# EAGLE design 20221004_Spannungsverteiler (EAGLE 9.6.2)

## Sheet 1 of 3: Anschlussklemmen
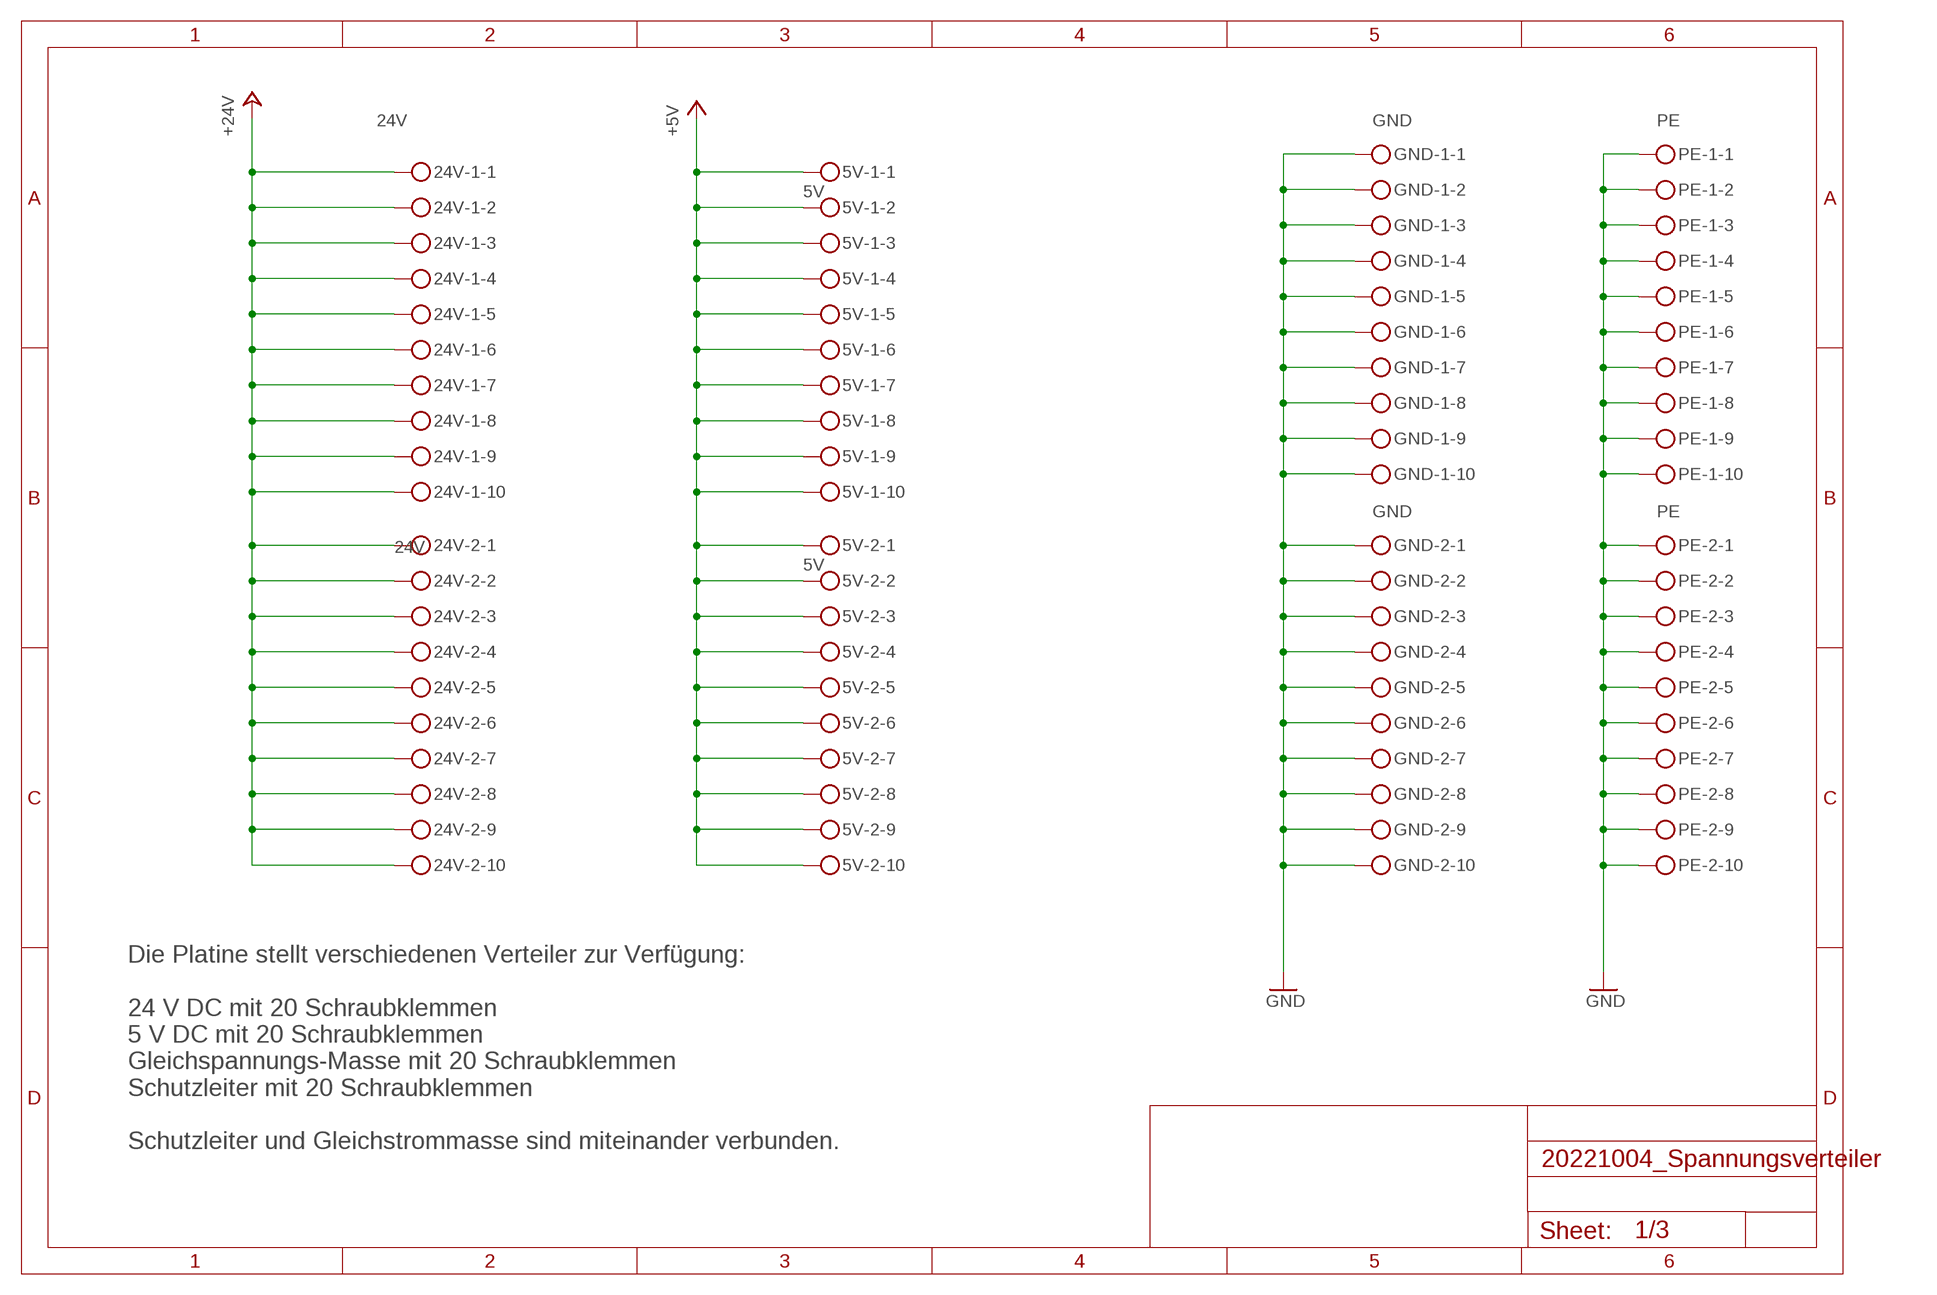
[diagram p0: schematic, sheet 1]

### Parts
5V-1  5V  MKDSN1,5/10-5,08  [MKDSN1,5/10-5,08]
5V-2  5V  MKDSN1,5/10-5,08  [MKDSN1,5/10-5,08]
24V-1  24V  MKDSN1,5/10-5,08  [MKDSN1,5/10-5,08]
24V-2  24V  MKDSN1,5/10-5,08  [MKDSN1,5/10-5,08]
GND-1  GND  MKDSN1,5/10-5,08  [MKDSN1,5/10-5,08]
GND-2  GND  MKDSN1,5/10-5,08  [MKDSN1,5/10-5,08]
PE-1  PE  MKDSN1,5/10-5,08  [MKDSN1,5/10-5,08]
PE-2  PE  MKDSN1,5/10-5,08  [MKDSN1,5/10-5,08]

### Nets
+5V: 5V-1.1 5V-1.2 5V-1.3 5V-1.4 5V-1.5 5V-1.6 5V-1.7 5V-1.8 5V-1.9 5V-1.10 5V-2.1 5V-2.2 5V-2.3 5V-2.4 5V-2.5 5V-2.6 5V-2.7 5V-2.8 5V-2.9 5V-2.10 ; also sheet 2,3
+24V: 24V-1.1 24V-1.2 24V-1.3 24V-1.4 24V-1.5 24V-1.6 24V-1.7 24V-1.8 24V-1.9 24V-1.10 24V-2.1 24V-2.2 24V-2.3 24V-2.4 24V-2.5 24V-2.6 24V-2.7 24V-2.8 24V-2.9 24V-2.10 ; also sheet 3
GND: GND-1.1 GND-1.2 GND-1.3 GND-1.4 GND-1.5 GND-1.6 GND-1.7 GND-1.8 GND-1.9 GND-1.10 GND-2.1 GND-2.2 GND-2.3 GND-2.4 GND-2.5 GND-2.6 GND-2.7 GND-2.8 GND-2.9 GND-2.10 PE-1.1 PE-1.2 PE-1.3 PE-1.4 PE-1.5 PE-1.6 PE-1.7 PE-1.8 PE-1.9 PE-1.10 PE-2.1 PE-2.2 PE-2.3 PE-2.4 PE-2.5 PE-2.6 PE-2.7 PE-2.8 PE-2.9 PE-2.10 ; also sheet 2,3

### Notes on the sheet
- Die Platine stellt verschiedenen Verteiler zur Verfügung:
  
  24 V DC mit 20 Schraubklemmen
  5 V DC mit 20 Schraubklemmen
  Gleichspannungs-Masse mit 20 Schraubklemmen
  Schutzleiter mit 20 Schraubklemmen
  
  Schutzleiter und Gleichstrommasse sind miteinander verbunden.

## Sheet 2 of 3: Schaltungen
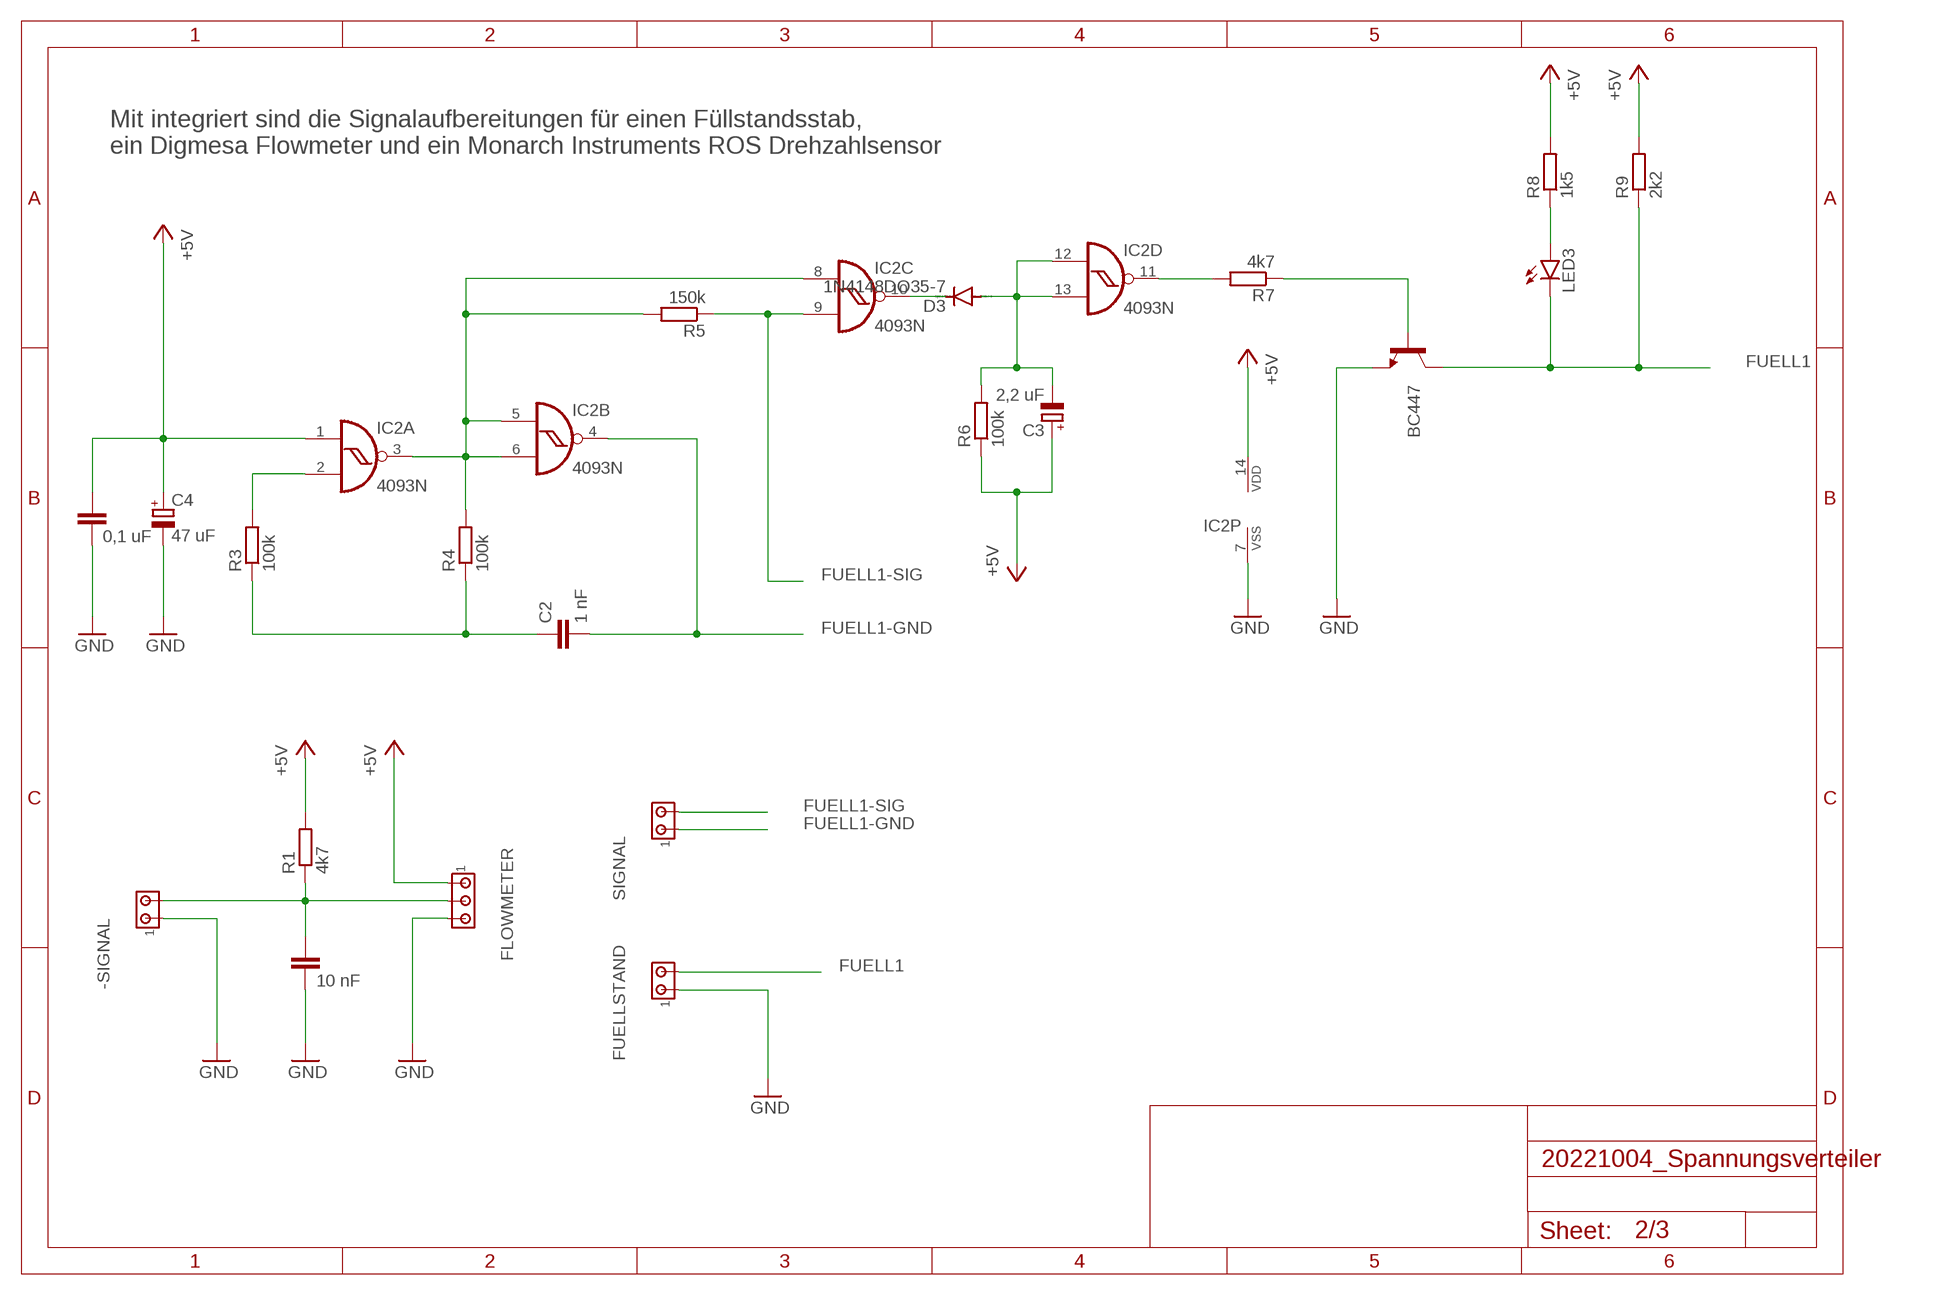
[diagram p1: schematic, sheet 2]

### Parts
-SIGNAL  MTA02-100  [10X02MTA]
C1  10 nF  C-EU050-024X044  [C050-024X044]
C2  1 nF  C-EU050-024X044  [C050-024X044]
C3  2,2 uF  CPOL-EUE2.5-7  [E2,5-7]
C4  47 uF  CPOL-EUE2.5-7  [E2,5-7]
C5  0,1 uF  C-EU050-024X044  [C050-024X044]
D3  1N4148DO35-7  [DO35-7]
FLOWMETER  MTA03-100  [10X03MTA]
FUELLSTAND  MTA02-100  [10X02MTA]
IC2  4093N  [DIL14]
LED3  LED3MM  [LED3MM]
Q1  BC447  [TO92-EBC]
R1  4k7  R-EU_0204/7  [0204/7]
R3  100k  R-EU_0204/7  [0204/7]
R4  100k  R-EU_0204/7  [0204/7]
R5  150k  R-EU_0204/7  [0204/7]
R6  100k  R-EU_0204/7  [0204/7]
R7  4k7  R-EU_0204/7  [0204/7]
R8  1k5  R-EU_0204/7  [0204/7]
R9  2k2  R-EU_0204/7  [0204/7]
SIGNAL  MTA02-100  [10X02MTA]

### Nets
+5V: C3.+ C4.+ C5.1 FLOWMETER.1 IC2.1(A:I0) IC2.14(P:VDD) R1.2 R6.1 R8.2 R9.2 ; also sheet 1,3
FUELL1: FUELLSTAND.2 LED3.K(C) Q1.C R9.1
FUELL1-GND: C2.2 IC2.4(B:O) SIGNAL.1
FUELL1-SIG: IC2.9(C:I1) R5.1 SIGNAL.2
GND: -SIGNAL.1 C1.2 C4.- C5.2 FLOWMETER.3 FUELLSTAND.1 IC2.7(P:VSS) Q1.E ; also sheet 1,3
N$2: -SIGNAL.2 C1.1 FLOWMETER.2 R1.1
N$3: IC2.2(A:I1) R3.2
N$4: IC2.3(A:O) IC2.5(B:I0) IC2.6(B:I1) IC2.8(C:I0) R4.2 R5.2
N$5: C2.1 R3.1 R4.1
N$6: D3.C IC2.10(C:O)
N$7: C3.- D3.A IC2.12(D:I0) IC2.13(D:I1) R6.2
N$8: IC2.11(D:O) R7.2
N$9: Q1.B R7.1
N$10: LED3.A R8.1

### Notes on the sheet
- Mit integriert sind die Signalaufbereitungen für einen Füllstandsstab, 
  ein Digmesa Flowmeter und ein Monarch Instruments ROS Drehzahlsensor

## Sheet 3 of 3: Spannungsregler
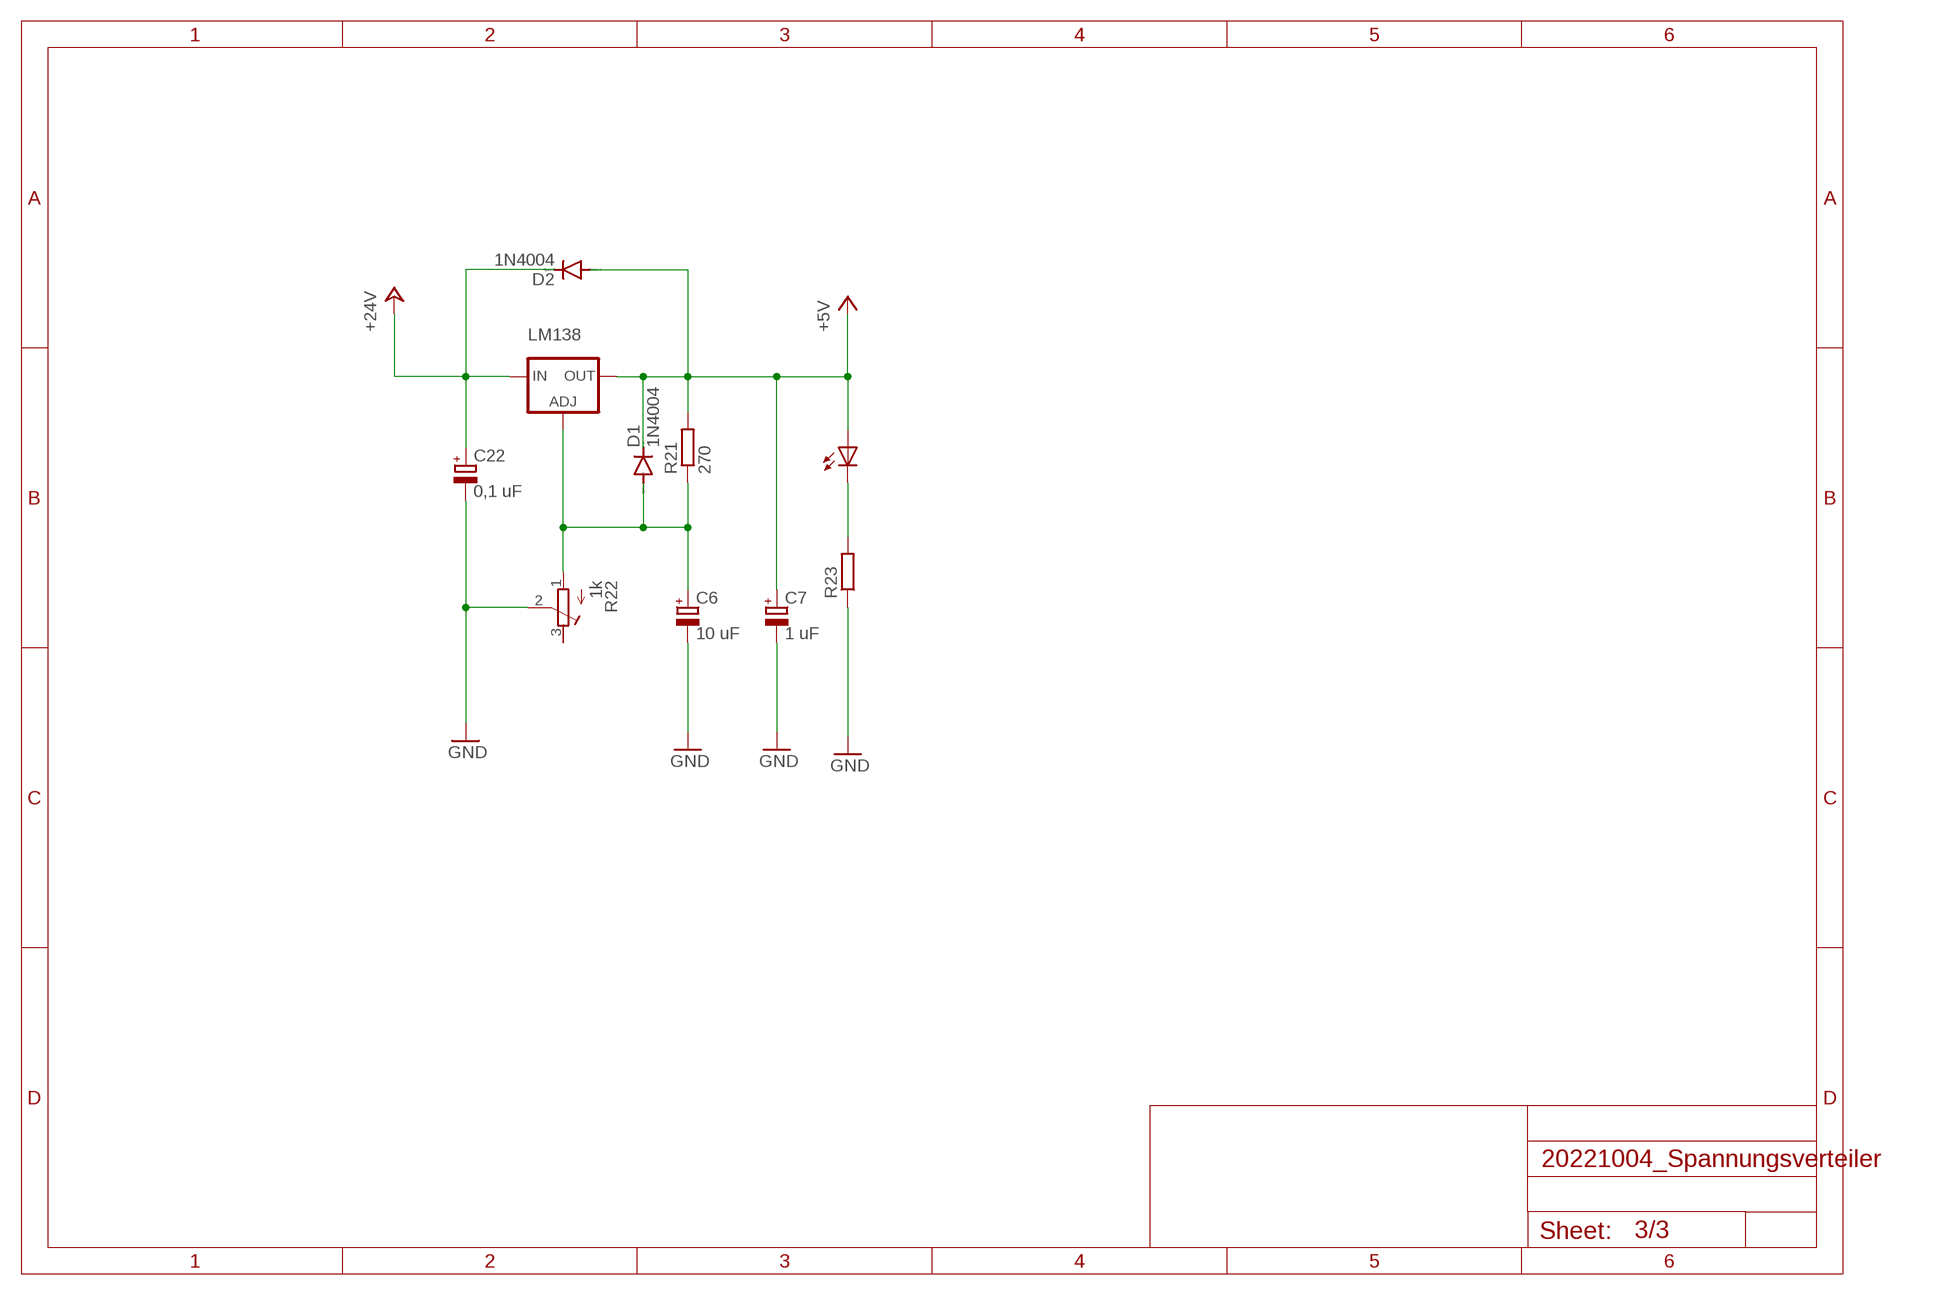
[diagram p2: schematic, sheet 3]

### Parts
C6  10 uF  CPOL-EUE2-5  [E2-5]
C7  1 uF  CPOL-EUE2-5  [E2-5]
C22  0,1 uF  CPOL-EUE2-5  [E2-5]
D1  1N4004  [DO41-10]
D2  1N4004  [DO41-10]
LED16  TLLG4400  [LED3MM]
LM138  LM138-TL  [TO220L1]
R21  270  R-EU_0204/7  [0204/7]
R22  1k  R-TRIMM64Y  [RTRIM64Y]
R23  R-EU_0204/7  [0204/7]

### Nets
+5V: C7.+ D1.C D2.A LED16.A LM138.2(OUT) R21.2 ; also sheet 1,2
+24V: C22.+ D2.C LM138.3(IN) ; also sheet 1
GND: C6.- C7.- C22.- R22.2(S) R23.1 ; also sheet 1,2
N$11: C6.+ D1.A LM138.1(ADJ) R21.1 R22.1(A)
N$14: LED16.K(C) R23.2
Unconnected: R22.3(E)

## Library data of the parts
5V-1 5V-2 24V-1 24V-2 GND-1 GND-2 PE-1 PE-2 = con-phoenix-508:MKDSN1,5/10-5,08: MKDSN 1,5/10-5,08 Printklemme Nennstrom: 13,5 A Nennspannung: 250 V Rastermaß: 5,08 mm Polzahl: 10 Anschlussart: Schraubanschluss Montage: Löten Anschlussrichtung Leiter/Platine: 0 ° Artikelnummer: 1729209 Source: http://eshop.phoenixcontact.com .. 1729209.pdf
-SIGNAL FUELLSTAND SIGNAL = con-amp:MTA02-100: AMP connector
C1 C2 C5 = resistor:C-EU: CAPACITOR, European symbol
C3 C4 C6 C7 C22 = resistor:CPOL-EU: POLARIZED CAPACITOR, European symbol
D1 D2 = diode:1N4004: DIODE
D3 = diode:1N4148: DIODE
FLOWMETER = con-amp:MTA03-100: AMP connector
IC2 = 40xx:4093: Quad 2-input NAND schmitt trigger
LED3 = led:LED: LED
LED16 = led:TLLG4400: Low Current (2mA) LED 3 mm Tinted Diffused Package color GREEN; MF: VISHAY SEMICONDUCTOR; OC_FARNELL: 1612435
LM138 = v-reg:LM138-TL: VOLTAGE REGULATOR
Q1 = transistor-npn:BC447*: NPN Transistor
R1 R3-R9 R21 R23 = resistor:R-EU_: RESISTOR, European symbol
R22 = resistor:R-TRIMM: Trimm resistor

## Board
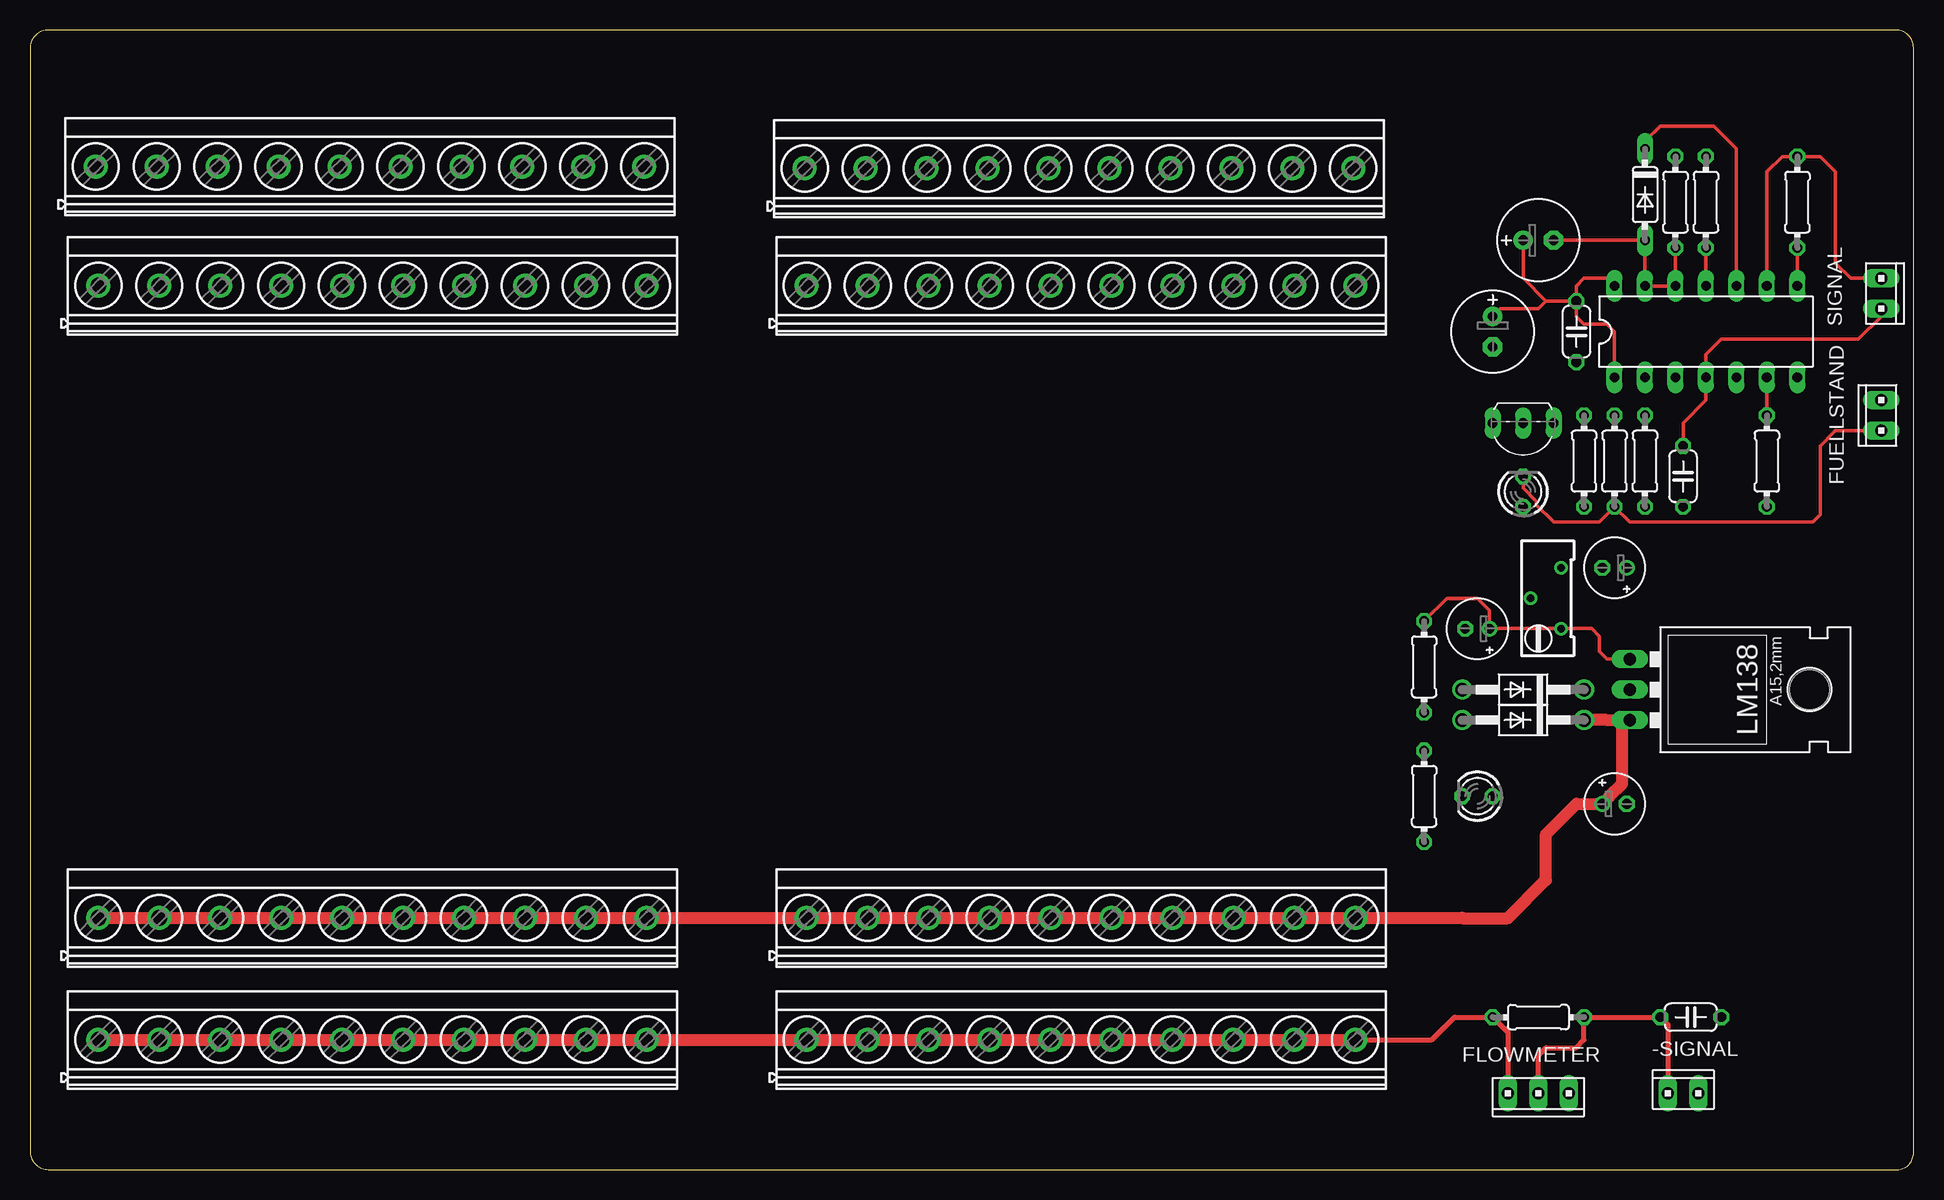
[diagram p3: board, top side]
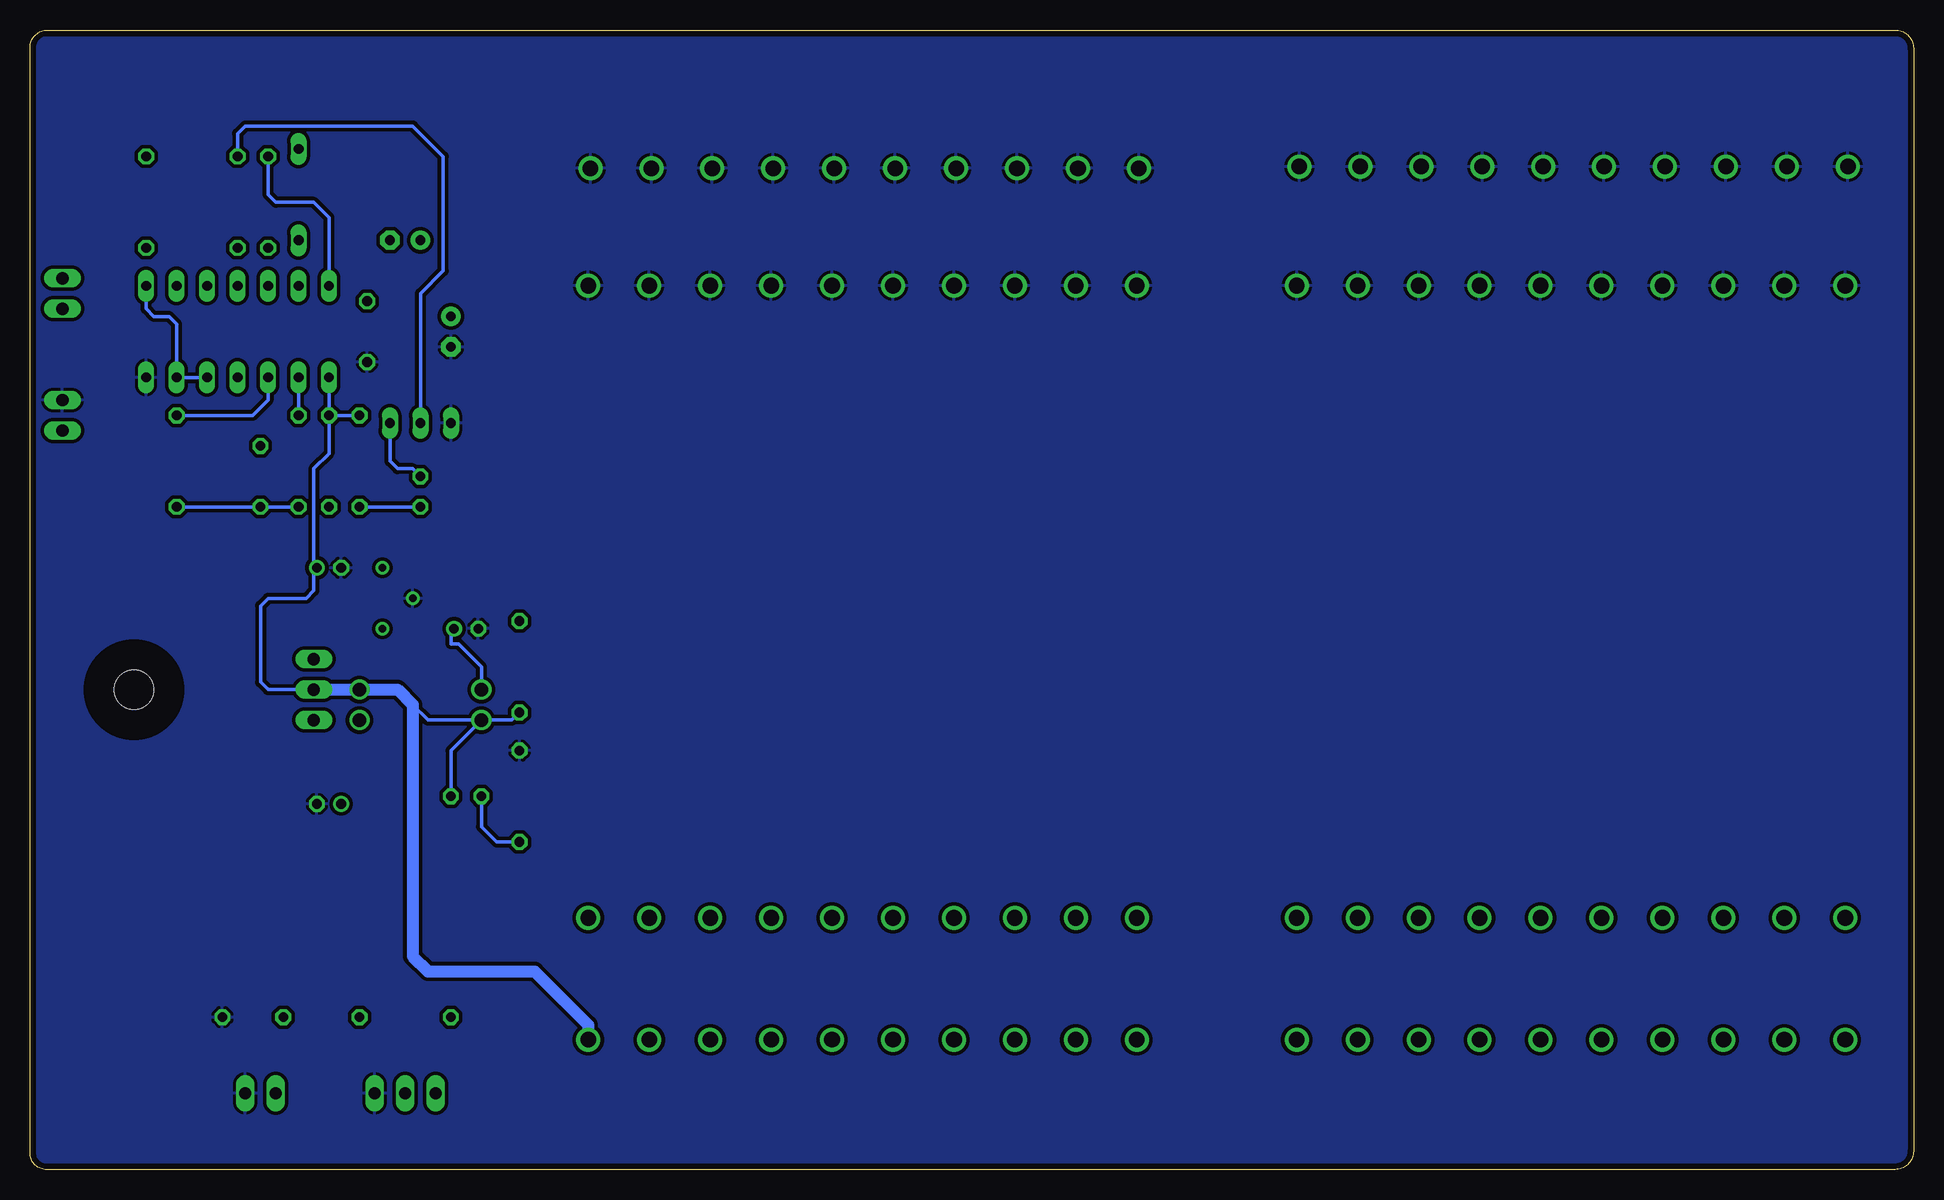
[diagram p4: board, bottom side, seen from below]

Size 157.01 x 95 mm. Coordinates in mm from the lower left corner, seen from the top.
Outline: 0,93.46 0,1.54 arc90 1.54,0 155.75,0 arc90 157,1.52 157,93.55 arc90 155.55,95 1.54,95 arc90 0,93.46
Copper layers (1*16): Top 0.035mm / dielectric 1.5mm / Bottom 0.035mm
Design rules "default *": minimum track width 12mil, minimum drill 0.35mm, track to track 12mil, track to pad 12mil, pad to pad 12mil, via to via 12mil, smd to smd 6mil, copper to edge 20mil, drill to drill 6mil, minimum pad ring 10mil, minimum via ring 8mil, stop-mask expansion 4mil, vias tented up to drill 0mil, thermal gap 10mil

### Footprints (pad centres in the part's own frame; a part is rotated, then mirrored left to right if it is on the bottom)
MKDSN1,5/10-5,08 = drill 1.3 pad 2: 1 -22.881,0.025; 2 -17.801,0.025; 3 -12.721,0.025; 4 -7.641,0.025; 5 -2.561,0.025; 6 2.519,0.025; 7 7.599,0.025; 8 12.679,0.025; 9 17.759,0.025; 10 22.839,0.025
10X02MTA = drill 1.016 long: 1 1.27,0; 2 -1.27,0
C050-024X044 = drill 0.813 octagon: 1 -2.54,0; 2 2.54,0
E2,5-7 = drill 0.813 pad 1.6: + -1.27,0 | drill 0.813 pad 1.6 octagon: - 1.27,0
E2-5 = drill 0.813 pad 1.27: + -1.016,0 | drill 0.813 pad 1.27 octagon: - 1.016,0
DO41-10 = drill 1.118: A 5.08,0; C -5.08,0
DO35-7 = drill 0.813 long: A 3.81,0; C -3.81,0
10X03MTA = drill 1.016 long: 1 2.54,0; 2 0,0; 3 -2.54,0
DIL14 = drill 0.813 long: 1 -7.62,-3.81; 2 -5.08,-3.81; 3 -2.54,-3.81; 4 0,-3.81; 5 2.54,-3.81; 6 5.08,-3.81; 7 7.62,-3.81; 8 7.62,3.81; 9 5.08,3.81; 10 2.54,3.81; 11 0,3.81; 12 -2.54,3.81; 13 -5.08,3.81; 14 -7.62,3.81
LED3MM = drill 0.813 octagon: A -1.27,0; K 1.27,0
TO220L1 = drill 1.016 long: 1 -2.54,-3.81; 2 0,-3.81; 3 2.54,-3.81 | hole 3.302: 0,11.176
TO92-EBC = drill 0.813 long: B 0,-1.27; C -2.54,-1.27; E 2.54,-1.27
0204/7 = drill 0.813 octagon: 1 -3.81,0; 2 3.81,0
RTRIM64Y = drill 0.61: 1 0,-2.54; 2 -2.54,0; 3 0,2.54

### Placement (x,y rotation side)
5V-1  28.57,10.79 0 top
5V-2  87.63,10.79 0 top
24V-1  28.57,20.95 0 top
24V-2  87.63,20.95 0 top
-SIGNAL  137.79,6.35 0 top
C1  138.43,12.7 0 top
C2  137.79,57.78 90 top
C3  125.73,77.47 0 top
C4  121.92,69.85 270 top
C5  128.91,69.85 270 top
C6  120.65,45.09 180 top
C7  132.08,50.16 180 top
C22  132.08,30.48 0 top
D1  124.46,40.01 180 top
D2  124.46,37.47 180 top
D3  134.62,81.28 270 top
FLOWMETER  125.73,6.35 180 top
FUELLSTAND  154.31,62.87 90 top
GND-1  87.63,73.66 0 top
GND-2  28.57,73.66 0 top
IC2  139.7,69.85 0 top
LED3  124.46,56.52 90 top
LED16  120.65,31.11 180 top
LM138  137.16,40.01 270 top
PE-1  87.45,83.44 0 top
PE-2  28.36,83.59 0 top
Q1  124.46,60.96 180 top
R1  125.73,12.7 180 top
R3  134.62,59.05 90 top
R4  144.78,59.05 90 top
R5  147.32,80.64 270 top
R6  137.16,80.64 270 top
R7  139.7,80.64 270 top
R8  129.54,59.05 90 top
R9  132.08,59.05 90 top
R21  116.2,41.91 270 top
R22  127.64,47.62 0 top
R23  116.2,31.11 270 top
SIGNAL  154.31,73.03 270 top

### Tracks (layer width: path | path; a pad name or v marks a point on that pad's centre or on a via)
+5V
  Top 0.305: IC2.14 131.44,74.3 129.54,74.3 128.91,73.66 C5.1 | C5.1 128.91,71.12 129.54,70.48 131.44,70.48 132.08,69.85 IC2.1 | C5.1 126.36,72.39 | C3.+ 124.46,74.3 126.36,72.39 | 126.36,72.39 125.73,71.75 122.56,71.75 C4.+
  Top 0.406: 5V-2.10 116.86,10.82 118.75,12.7 R1.2 123.19,11.43 FLOWMETER.1
  Top 1.016: 5V-1.1 5V-1.2 5V-1.3 5V-1.4 5V-1.5 5V-1.6 5V-1.7 5V-1.8 5V-1.9 5V-1.10 5V-2.1 5V-2.2 5V-2.3 5V-2.4 5V-2.5 5V-2.6 5V-2.7 5V-2.8 5V-2.9 5V-2.10
  Bottom 0.305: 125.09,38.73 123.83,37.47 D2.A | D2.A 121.92,34.92 LED16.A | D2.A 116.84,37.47 R21.2 | R9.2 IC2.1 | R9.2 R8.2 | IC2.14 132.08,79.38 133.35,80.64 136.53,80.64 137.16,81.28 R6.1 | R9.2 132.08,59.69 133.35,58.42 133.35,50.42 C7.+ 133.35,49.91 133.35,48.26 133.99,47.62 137.16,47.62 137.79,46.99 137.79,40.64 137.16,40.01 LM138.2
  Bottom 1.016: LM138.2 D1.C 126.36,40.01 125.09,38.73 125.09,17.78 123.83,16.51 114.94,16.51 110.47,12.04 5V-2.10
+24V
  Top 1.016: 24V-1.1 24V-1.2 24V-1.3 24V-1.4 24V-1.5 24V-1.6 24V-1.7 24V-1.8 24V-1.9 24V-1.10 24V-2.1 24V-2.2 24V-2.3 24V-2.4 24V-2.5 24V-2.6 24V-2.7 24V-2.8 24V-2.9 24V-2.10 119.36,20.98 119.38,20.95 123.19,20.95 126.36,24.13 126.36,27.94 128.91,30.48 C22.+ 131.62,31.04 131.62,31.09 132.72,32.18 132.72,37.47 | 132.72,37.47 131.44,37.47 D2.C | LM138.3 132.72,37.47
FUELL1
  Top 0.305: FUELLSTAND.2 150.5,61.59 149.22,60.33 149.22,54.61 148.59,53.98 133.35,53.98 R9.1 130.81,53.98 127,53.98 125.58,55.4 125.58,55.71 124.46,56.83 LED3.K
  Bottom 0.305: LED3.K 125.09,58.42 126.36,58.42 127,59.05 Q1.C
FUELL1-GND
  Top 0.305: C2.2 137.79,62.23 139.7,64.14 IC2.4 139.7,67.94 140.97,69.22 152.4,69.22 154.31,71.12 SIGNAL.1
FUELL1-SIG
  Top 0.305: IC2.9 144.78,83.19 146.05,84.45 R5.1 149.22,84.45 150.5,83.19 150.5,75.56 151.76,74.3 SIGNAL.2
GND
  pour Bottom: -1.27,95.89 158.12,95.89 158.12,-0.64 0,-0.64 -0.64,0 -0.64,95.25
N$2
  Top 0.406: FLOWMETER.2 125.73,9.53 126.36,10.16 128.91,10.16 129.54,10.79 R1.1 C1.1 136.53,12.06 -SIGNAL.2
N$3
  Bottom 0.305: R3.2 IC2.2
N$4
  Top 0.305: IC2.6 R4.2 | IC2.8 R5.2
  Bottom 0.305: IC2.3 137.16,64.14 138.43,62.87 R4.2 | IC2.5 IC2.6 144.78,70.48 145.41,71.12 146.69,71.12 147.32,71.75 IC2.8
N$5
  Bottom 0.305: R3.1 C2.1 R4.1
N$6
  Top 0.305: D3.C 134.62,85.72 135.89,87 140.34,87 142.24,85.09 IC2.10
N$7
  Top 0.305: R6.2 IC2.12 IC2.13 D3.A C3.-
N$8
  Top 0.305: R7.2 IC2.11
N$9
  Bottom 0.305: R7.1 139.7,86.36 139.06,87 125.09,87 122.56,84.45 122.56,74.93 124.46,73.03 Q1.B
N$10
  Bottom 0.305: LED3.A R8.1
N$11
  Top 0.305: LM138.1 131.44,42.55 130.81,43.18 130.81,44.45 130.18,45.09 R22.1 C6.+ 121.67,46.61 120.65,47.62 118.11,47.62 R21.1
  Bottom 0.305: D1.A 119.38,41.91 121.28,43.81 121.92,43.81 121.92,44.83 121.79,44.96 C6.+
N$14
  Bottom 0.305: LED16.K 119.38,28.57 118.11,27.3 R23.2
